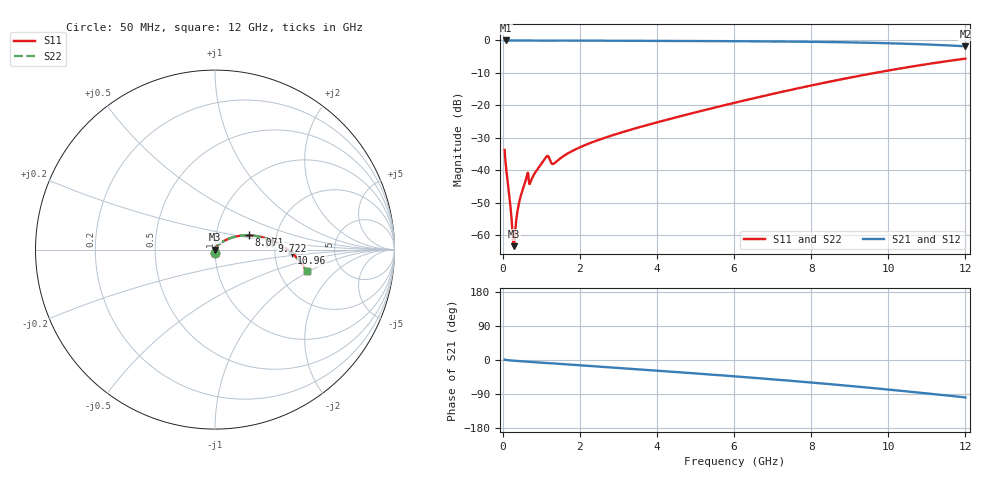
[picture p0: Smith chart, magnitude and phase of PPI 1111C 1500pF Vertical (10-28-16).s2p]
# GHz S MA R 50
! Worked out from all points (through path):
!   1601 points, 50 MHz to 12 GHz, reference 50 ohm
!   highest |S21| = 0.00 dB at 94.81 MHz (marker M1); lowest = -1.8 dB at 12 GHz (marker M2)
!   group delay of S21, straight-line fit = 22.4 ps
!   lowest |S11| = -63.4 dB at 289 MHz (marker M3), VSWR 1.00, Z = 50.1 - j0.00103 ohm
!   |S11| at or under -10 dB: start of sweep to 9.655 GHz
!   |S22| runs from -63.4 to -5.6 dB; largest |S21 - S12| = 0
!   S11 on the Smith chart (normalised r, x): 50 MHz: 1.00, -0.04; 8.071 GHz: 1.45, +0.24; 9.722 GHz: 1.91, +0.22; 10.96 GHz: 2.49, -0.12; 12 GHz: 2.87, -0.93
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0.05  0.02053 -88.1  0.9994 0.9  0.9994 0.9  0.02053 -88.1
0.0948125  0.009994 -87.8  0.9996 -0.0  0.9996 -0.0  0.009994 -87.8
0.1769688  0.00379 -83.3  0.9995 -0.9  0.9995 -0.9  0.00379 -83.3
0.2441875  0.001384 -65.5  0.9994 -1.5  0.9994 -1.5  0.001384 -65.5
0.2665938  0.0008706 -44.2  0.9993 -1.7  0.9993 -1.7  0.0008706 -44.2
0.289  0.0006776 -0.9  0.9993 -1.8  0.9993 -1.8  0.0006776 -0.9
0.3263437  0.001183 49.1  0.9992 -2.1  0.9992 -2.1  0.001183 49.1
0.3860938  0.002386 66.6  0.9991 -2.6  0.9991 -2.6  0.002386 66.6
0.438375  0.003426 70.8  0.999 -3.0  0.999 -3.0  0.003426 70.8
0.6101562  0.007446 71.3  0.9981 -4.3  0.9981 -4.3  0.007446 71.3
0.7445938  0.007122 68.4  0.9979 -5.1  0.9979 -5.1  0.007122 68.4
1.132969  0.01619 60.1  0.9938 -8.1  0.9938 -8.1  0.01619 60.1
1.327156  0.01268 55.9  0.9945 -9.1  0.9945 -9.1  0.01268 55.9
2.044156  0.02315 60.8  0.9937 -14.3  0.9937 -14.3  0.02315 60.8
4.038312  0.05543 47.5  0.9848 -28.4  0.9848 -28.4  0.05543 47.5
6.025  0.11 36.3  0.9737 -43.2  0.9737 -43.2  0.11 36.3
8.019156  0.2034 23.0  0.9526 -59.6  0.9526 -59.6  0.2034 23.0
8.071438  0.2065 22.6  0.9518 -60.0  0.9518 -60.0  0.2065 22.6
9.722031  0.3215 9.1  0.9151 -75.3  0.9151 -75.3  0.3215 9.1
10.01331  0.3452 6.4  0.9059 -78.1  0.9059 -78.1  0.3452 6.4
10.96184  0.4278 -2.5  0.8683 -87.8  0.8683 -87.8  0.4278 -2.5
12  0.5246 -13.0  0.813 -98.7  0.813 -98.7  0.5246 -13.0
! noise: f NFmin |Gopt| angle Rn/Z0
0.05  0.0004088  0.8773  0.3296  0.0007204
1.372  0.007862  0.8302  8.733  0.009702
2.701  0.01455  0.8228  17.07  0.01686
4.031  0.02225  0.8304  25.21  0.02634
5.36  0.02928  0.8337  33.07  0.03418
6.682  0.03576  0.8365  40.56  0.04073
8.012  0.04206  0.8403  47.71  0.04674
9.341  0.04841  0.8456  54.46  0.05278
10.67  0.05508  0.8525  60.82  0.05937
12  0.06231  0.8608  66.77  0.06704
